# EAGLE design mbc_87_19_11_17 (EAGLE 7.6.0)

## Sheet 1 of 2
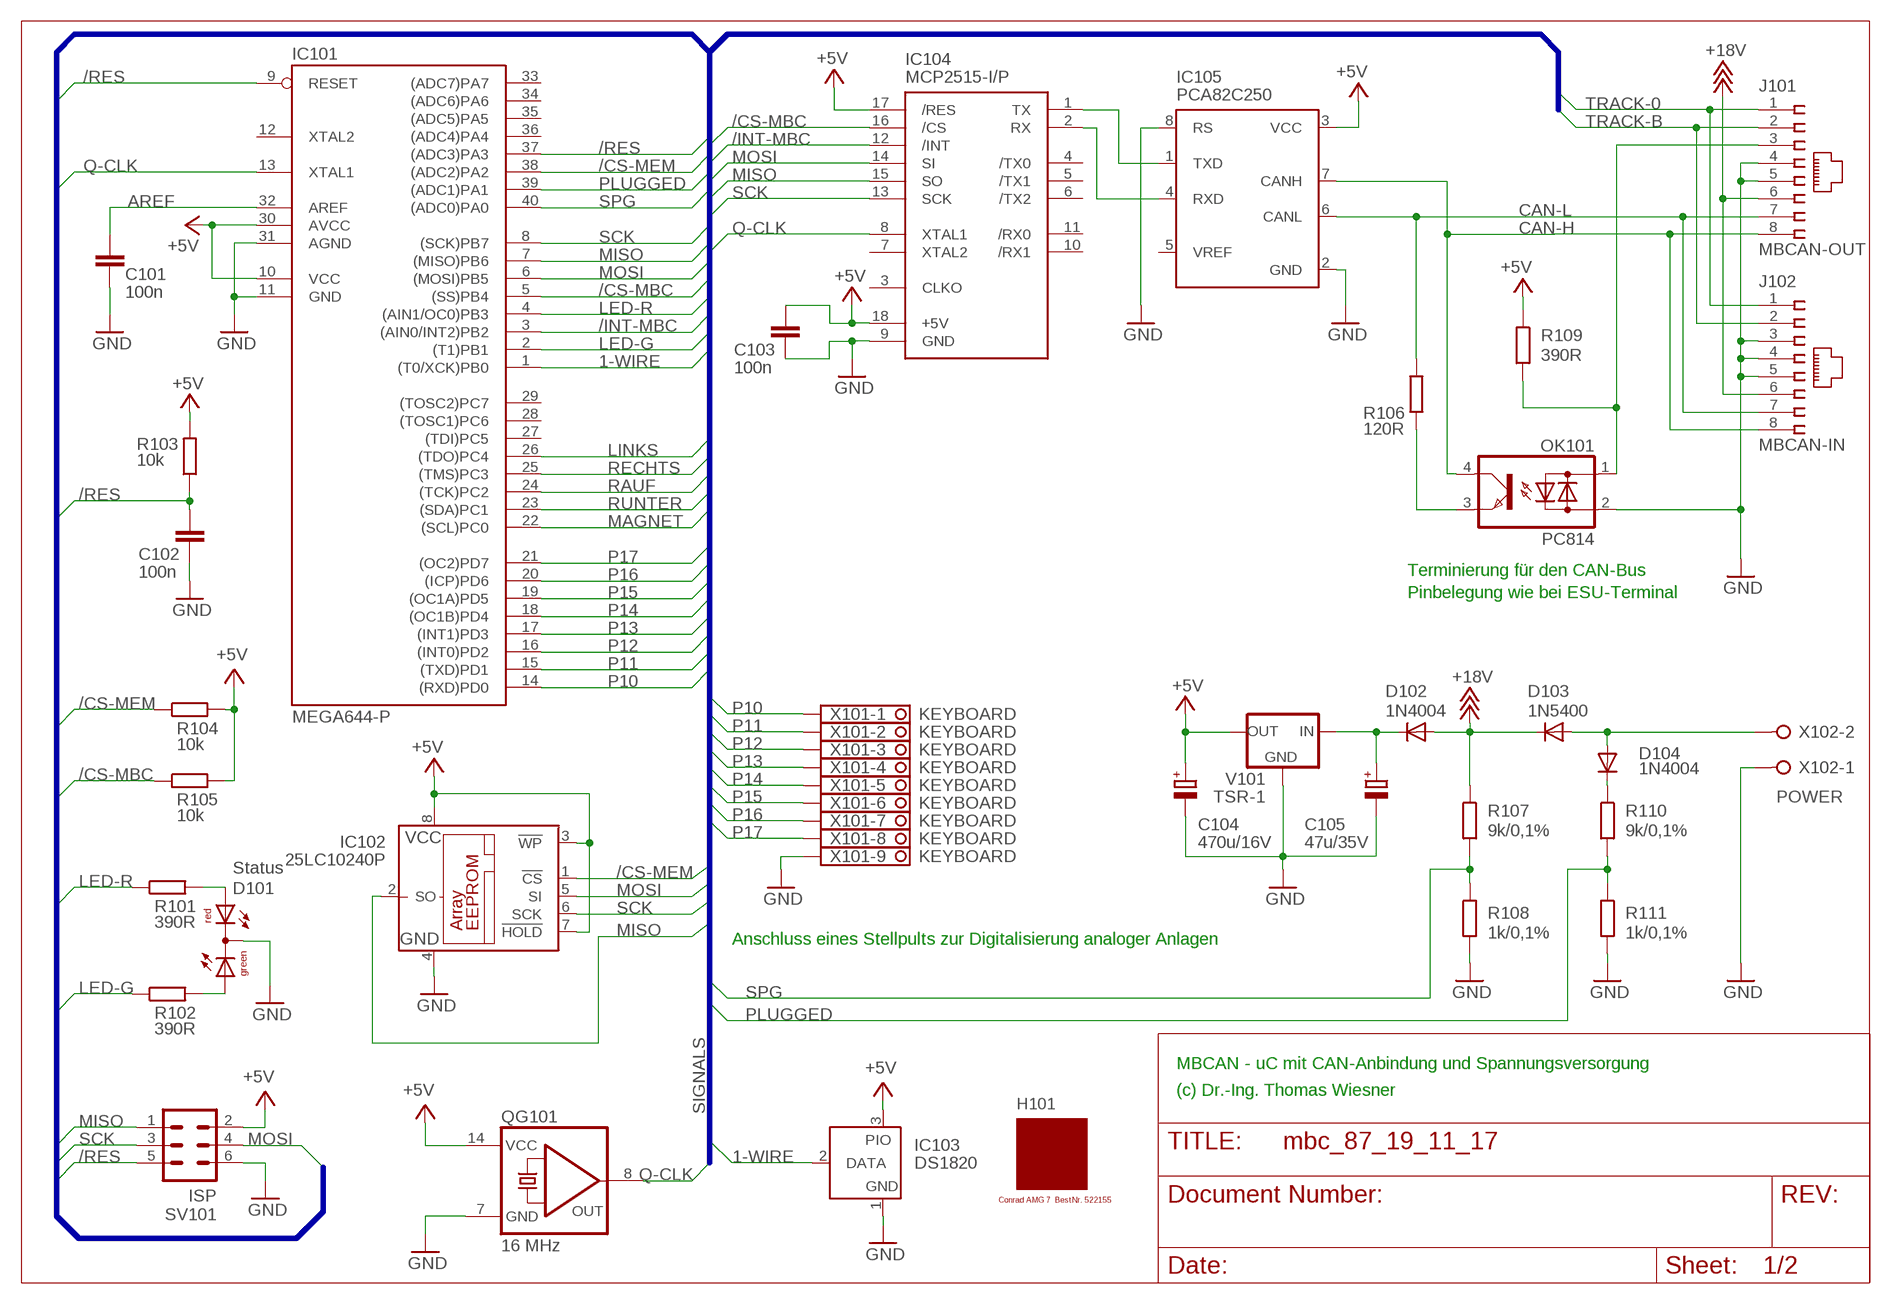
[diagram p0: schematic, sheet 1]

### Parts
C101  100n  C-EU025-025X050  [C025-025X050]
C102  100n  C-EU025-025X050  [C025-025X050]
C103  100n  C-EU025-025X050  [C025-025X050]
C104  470u/16V  CPOL-EUE3.5-8  [E3,5-8]
C105  47u/35V  CPOL-EUE2.5-7  [E2,5-7]
D101  Status  DUOLED5MM  [DUOLED5MM]
D102  1N4004  [DO41-10]
D103  1N5400  [DO201-15]
D104  1N4004  [DO41-10]
H101  MODULGEHÄUSE-AMG-7  [MODULGEHÄUSE-1]
IC101  MEGA644-P  MEGA323-P  [DIL40]
IC102  25LC10240P  25LC040P  [DIL8]
IC103  DS1820  DS2405  [TO92-]
IC104  MCP2515-I/P  MCP2510-I/P  [DIL18]
IC105  PCA82C250  [DIL08]
J101  MBCAN-OUT  215877-4  [215877-4]
J102  MBCAN-IN  215877-4  [215877-4]
OK101  PC814  [DIL04]
QG101  16 MHz  QG5860  [DIL14S]
R101  390R  R-EU_0207/10  [0207/10]
R102  390R  R-EU_0207/10  [0207/10]
R103  10k  R-EU_0207/10  [0207/10]
R104  10k  R-EU_0207/10  [0207/10]
R105  10k  R-EU_0207/10  [0207/10]
R106  120R  R-EU_0207/10  [0207/10]
R107  9k/0,1%  R-EU_0207/10  [0207/10]
R108  1k/0,1%  R-EU_0207/10  [0207/10]
R109  390R  R-EU_0207/10  [0207/10]
R110  9k/0,1%  R-EU_0207/10  [0207/10]
R111  1k/0,1%  R-EU_0207/10  [0207/10]
SV101  ISP  ML6  [ML6]
V101  TSR-1  [TRACO-TSR-1]
X101  KEYBOARD  1751316  [1751316]
X102  POWER  W237-02P  [W237-132]

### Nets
1-WIRE: IC101.1((T0/XCK)PB0) IC103.2(DATA)
+5V: C103.1 C104.+ IC101.10(VCC) IC101.30(AVCC) IC102.3(!WP) IC102.7(!HOLD) IC102.8(VCC) IC103.3(PIO) IC104.17(/RES) IC104.18(+5V) IC105.3(VCC) QG101.14(VCC) R103.2 R104.2 R105.2 R109.1 SV101.2 V101.OUT ; also sheet 2
+18V: D102.A D103.C J101.6 J102.6 R107.1
/CS-MBC: IC101.5((SS)PB4) IC104.16(/CS) R105.1
/CS-MEM: IC101.38((ADC2)PA2) IC102.1(!CS) R104.1
/INT-MBC: IC101.3((AIN0/INT2)PB2) IC104.12(/INT)
/RES: C102.1 IC101.9(RESET) IC101.37((ADC3)PA3) R103.1 SV101.5
AREF: C101.1 IC101.32(AREF)
CAN-H: IC105.7(CANH) J101.8 J102.8 OK101.4(C)
CAN-L: IC105.6(CANL) J101.7 J102.7 R106.2
GND: C101.2 C102.2 C103.2 C104.- C105.- D101.K(C) IC101.11(GND) IC101.31(AGND) IC102.4(GND) IC103.1(GND) IC104.9(GND) IC105.2(GND) IC105.8(RS) J101.4 J101.5 J102.3 J102.4 J102.5 OK101.2(AC2) QG101.7(GND) R108.2 R111.2 SV101.6 V101.GND X101.9 X102.1 ; also sheet 2
LED-G: IC101.2((T1)PB1) R102.1
LED-R: IC101.4((AIN1/OC0)PB3) R101.1
LINKS: IC101.26((TDO)PC4) ; also sheet 2
MAGNET: IC101.22((SCL)PC0) ; also sheet 2
MISO: IC101.7((MISO)PB6) IC102.2(SO) IC104.15(SO) SV101.1
MOSI: IC101.6((MOSI)PB5) IC102.5(SI) IC104.14(SI) SV101.4
N$1: IC104.1(TX) IC105.1(TXD)
N$2: IC104.2(RX) IC105.4(RXD)
N$3: OK101.3(E) R106.1
N$4: J101.3 OK101.1(AC1) R109.2
N$5: D104.C R110.1
N$6: C105.+ D102.C V101.IN
N$9: D101.AR R101.2
N$13: D101.AG R102.2
P10: IC101.14((RXD)PD0) X101.1
P11: IC101.15((TXD)PD1) X101.2
P12: IC101.16((INT0)PD2) X101.3
P13: IC101.17((INT1)PD3) X101.4
P14: IC101.18((OC1B)PD4) X101.5
P15: IC101.19((OC1A)PD5) X101.6
P16: IC101.20((ICP)PD6) X101.7
P17: IC101.21((OC2)PD7) X101.8
PLUGGED: IC101.39((ADC1)PA1) R110.2 R111.1
Q-CLK: IC101.13(XTAL1) IC104.8(XTAL1) QG101.8(OUT)
RAUF: IC101.24((TCK)PC2) ; also sheet 2
RECHTS: IC101.25((TMS)PC3) ; also sheet 2
RUNTER: IC101.23((SDA)PC1) ; also sheet 2
SCK: IC101.8((SCK)PB7) IC102.6(SCK) IC104.13(SCK) SV101.3
SPG: IC101.40((ADC0)PA0) R107.2 R108.1
TRACK-0: J101.1 J102.1
TRACK-B: J101.2 J102.2
V-NETZTEIL: D103.A D104.A X102.2
Unconnected: IC101.12(XTAL2) IC101.27((TDI)PC5) IC101.28((TOSC1)PC6) IC101.29((TOSC2)PC7) IC101.33((ADC7)PA7) IC101.34((ADC6)PA6) IC101.35((ADC5)PA5) IC101.36((ADC4)PA4) IC104.3(CLKO) IC104.4(/TX0) IC104.5(/TX1) IC104.6(/TX2) IC104.7(XTAL2) IC104.10(/RX1) IC104.11(/RX0) IC105.5(VREF)

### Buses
SIGNALS

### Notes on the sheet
- Terminierung für den CAN-Bus
- Pinbelegung wie bei ESU-Terminal
- Anschluss eines Stellpults zur Digitalisierung analoger Anlagen
- MBCAN - uC mit CAN-Anbindung und Spannungsversorgung
- (c) Dr.-Ing. Thomas Wiesner

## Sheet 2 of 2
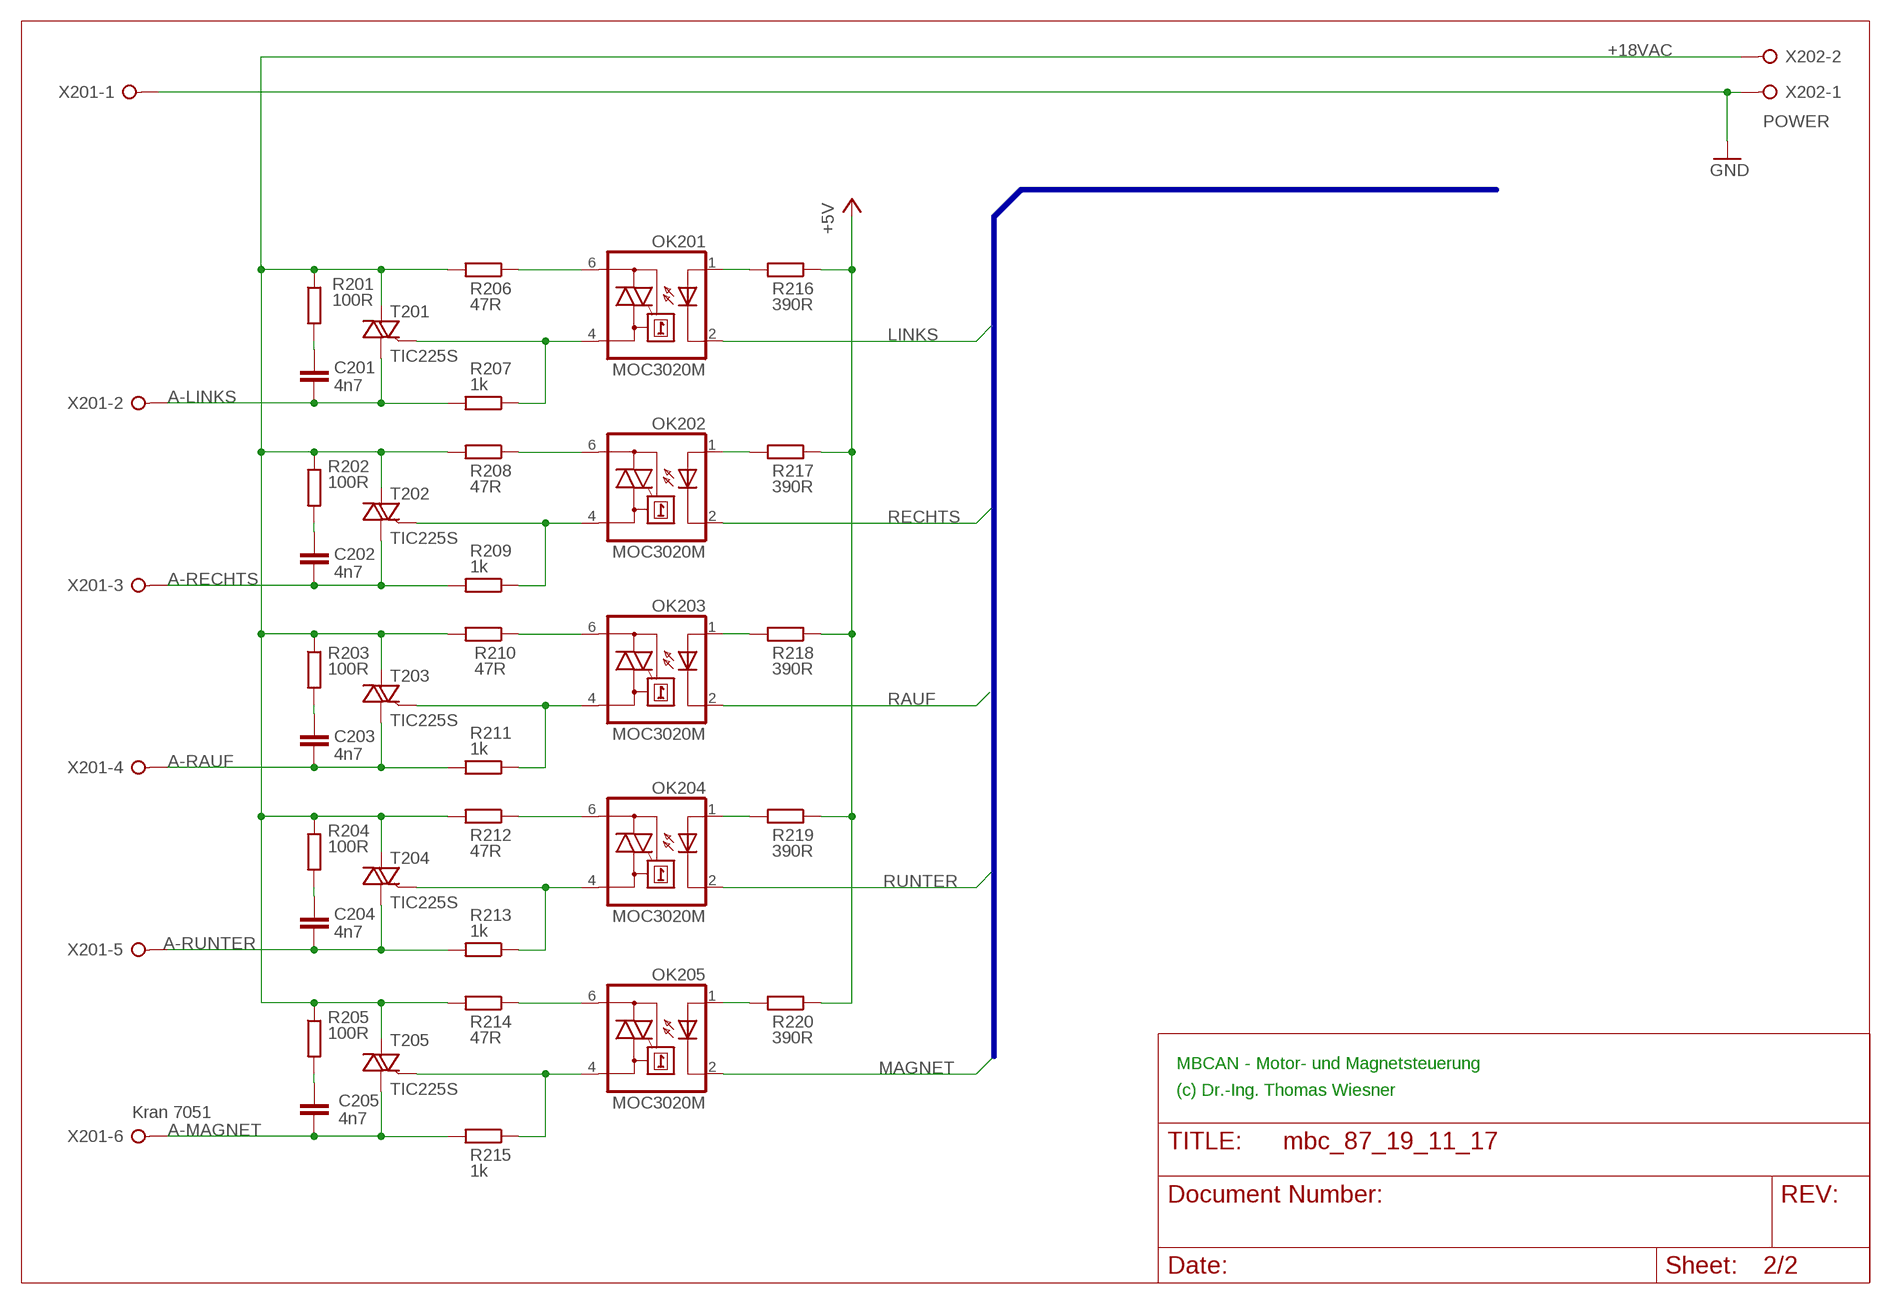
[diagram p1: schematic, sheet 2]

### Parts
C201  4n7  C-EU025-025X050  [C025-025X050]
C202  4n7  C-EU025-025X050  [C025-025X050]
C203  4n7  C-EU025-025X050  [C025-025X050]
C204  4n7  C-EU025-025X050  [C025-025X050]
C205  4n7  C-EU025-025X050  [C025-025X050]
OK201  MOC3020M  [DIL06]
OK202  MOC3020M  [DIL06]
OK203  MOC3020M  [DIL06]
OK204  MOC3020M  [DIL06]
OK205  MOC3020M  [DIL06]
R201  100R  R-EU_0207/10  [0207/10]
R202  100R  R-EU_0207/10  [0207/10]
R203  100R  R-EU_0207/10  [0207/10]
R204  100R  R-EU_0207/10  [0207/10]
R205  100R  R-EU_0207/10  [0207/10]
R206  47R  R-EU_0207/10  [0207/10]
R207  1k  R-EU_0207/10  [0207/10]
R208  47R  R-EU_0207/10  [0207/10]
R209  1k  R-EU_0207/10  [0207/10]
R210  47R  R-EU_0207/10  [0207/10]
R211  1k  R-EU_0207/10  [0207/10]
R212  47R  R-EU_0207/10  [0207/10]
R213  1k  R-EU_0207/10  [0207/10]
R214  47R  R-EU_0207/10  [0207/10]
R215  1k  R-EU_0207/10  [0207/10]
R216  390R  R-EU_0207/10  [0207/10]
R217  390R  R-EU_0207/10  [0207/10]
R218  390R  R-EU_0207/10  [0207/10]
R219  390R  R-EU_0207/10  [0207/10]
R220  390R  R-EU_0207/10  [0207/10]
T201  TIC225S  [TO220DS]
T202  TIC225S  [TO220DS]
T203  TIC225S  [TO220DS]
T204  TIC225S  [TO220DS]
T205  TIC225S  [TO220DS]
X201  Kran 7051  W237-06P  [W237-6P]
X202  POWER  W237-02P  [W237-132]

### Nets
+5V: R216.1 R217.1 R218.1 R219.1 R220.1 ; also sheet 1
+18VAC: R201.1 R202.1 R203.1 R204.1 R205.1 R206.2 R208.2 R210.2 R212.2 R214.2 T201.A2 T202.A2 T203.A2 T204.A2 T205.A2 X202.2
A-LINKS: C201.2 R207.2 T201.A1 X201.2
A-MAGNET: C205.2 R215.2 T205.A1 X201.6
A-RAUF: C203.2 R211.2 T203.A1 X201.4
A-RECHTS: C202.2 R209.2 T202.A1 X201.3
A-RUNTER: C204.2 R213.2 T204.A1 X201.5
GND: X201.1 X202.1 ; also sheet 1
LINKS: OK201.2(C) ; also sheet 1
MAGNET: OK205.2(C) ; also sheet 1
N$7: OK201.1(A) R216.2
N$10: OK201.4(A1) R207.1 T201.G
N$11: OK201.6(A2) R206.1
N$12: OK202.1(A) R217.2
N$15: C201.1 R201.2
N$17: OK202.4(A1) R209.1 T202.G
N$18: OK202.6(A2) R208.1
N$20: C202.1 R202.2
N$21: OK203.1(A) R218.2
N$23: OK203.4(A1) R211.1 T203.G
N$24: OK203.6(A2) R210.1
N$26: C203.1 R203.2
N$27: OK204.1(A) R219.2
N$29: OK204.4(A1) R213.1 T204.G
N$30: OK204.6(A2) R212.1
N$32: C204.1 R204.2
N$33: OK205.1(A) R220.2
N$35: OK205.4(A1) R215.1 T205.G
N$36: OK205.6(A2) R214.1
N$38: C205.1 R205.2
RAUF: OK203.2(C) ; also sheet 1
RECHTS: OK202.2(C) ; also sheet 1
RUNTER: OK204.2(C) ; also sheet 1

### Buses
B$1

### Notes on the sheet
- MBCAN - Motor- und Magnetsteuerung
- (c) Dr.-Ing. Thomas Wiesner

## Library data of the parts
C101-C103 = rcl:C-EU: CAPACITOR, European symbol
C104 C105 = rcl:CPOL-EU: POLARIZED CAPACITOR, European symbol
C201-C205 = resistor:C-EU: CAPACITOR, European symbol
D101 = led:DUOLED5MM: DUO LED 2 colors, 5 mm, round
D102 D104 = diode:1N4004: DIODE
D103 = diode:1N5400: DIODE
H101 = mbc:MODULGEHÄUSE-AMG-7: Gehäuse
IC101 = atmel:MEGA323-P: MICROCONTROLLER 32 Kbytes FLASH 2 Kbytes SRAM 1 Kbytes EEPROM USART 8-channel 10 bit ADC Source: avr.lbr; OC_FARNELL: unknown; OC_NEWARK: unknown
IC102 = microchip:25*: Serial EEPROM 4K/ 8K , SPI bus; MF: MICROCHIP; MPN: 25LC040/P; OC_FARNELL: 9758100; OC_NEWARK: 96K4091
IC103 = maxim:DS2405: Addressable Switch DALLAS Semiconductor; MF: DALLAS SEMICONDUCTOR; MPN: DS2405; OC_FARNELL: 1188025; OC_NEWARK: 06F4645
IC104 = mbc:MCP2510: BASIC-CAN 2.0a Controller Stand-alone CAN controller von Microchip
IC105 = micro-philips:PCA82C250: CAN CONTROLLER INTERFACE; OC_FARNELL: 3692358; OC_NEWARK: unknown
J101 J102 = con-amp:215877-4: AMP connector
OK101 = optocoupler:PC814: SHARP OPTO COUPLER; OC_FARNELL: 9707662; OC_NEWARK: unknown
OK201-OK205 = optocoupler:MOC30*M: RANDOM-PHASE OPTOISOLATORS TRIAC DRIVER OUTPUT Source: http://www.fairchildsemi.com MOC3020-M.pdf; MF: FAIRCHILD SEMICONDUCTOR; MPN: MOC3020-M; OC_FARNELL: 1505425; OC_NEWARK: 72K8895
QG101 = crystal:QG5860: CRYSTAL RESONATOR; OC_FARNELL: unknown; OC_NEWARK: unknown
R101-R111 R201-R220 = resistor:R-EU_: RESISTOR, European symbol
SV101 = con-ml:ML6: HARTING; OC_FARNELL: unknown; OC_NEWARK: unknown
T201-T205 = triac:TIC225S: TRIAC
V101 = mbc:TSR-1: Spannungsregler Hersteller: TRACO Typ: TSR-1 5V: TSR 1-2450 Spg: 5V Strom: 1A Reichelt TSR 1-2450
X101 = con-phoenix-350:1751316: MKDS 1/ 9-3,5 Printklemme Nennstrom: 10 A Bemessungsspannung: 160 V Raster: 3,5 mm Polzahl: 9 Montageart: Löten Anschlussart: Schraubanschluss Anschlussrichtung vom Leiter zur Platine: 0° Source: http://eshop.phoenixcontact.com .. 1751316.pdf; OC_FARNELL: unknown; OC_NEWARK: unknown
X102 X202 = con-wago-508:W237-02P: WAGO SREW CLAMP; OC_FARNELL: unknown; OC_NEWARK: unknown
X201 = con-wago-508:W237-06P: WAGO SREW CLAMP; OC_FARNELL: unknown; OC_NEWARK: unknown

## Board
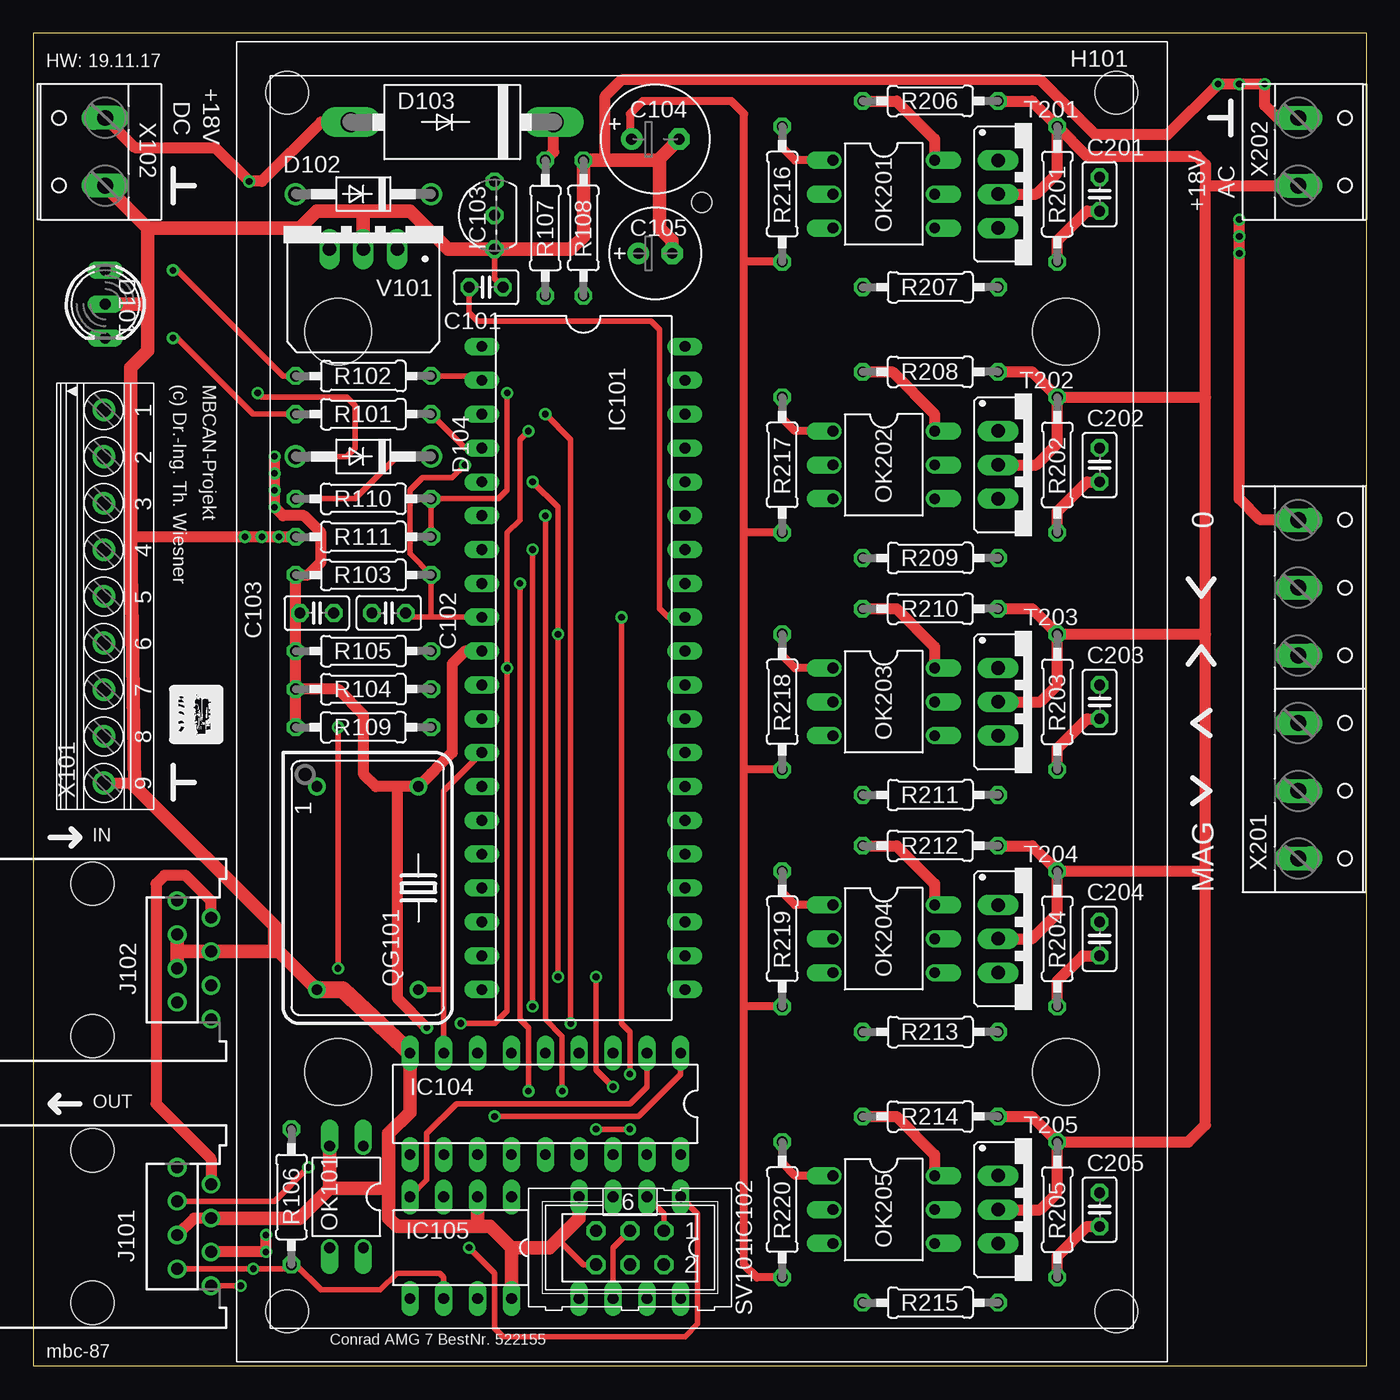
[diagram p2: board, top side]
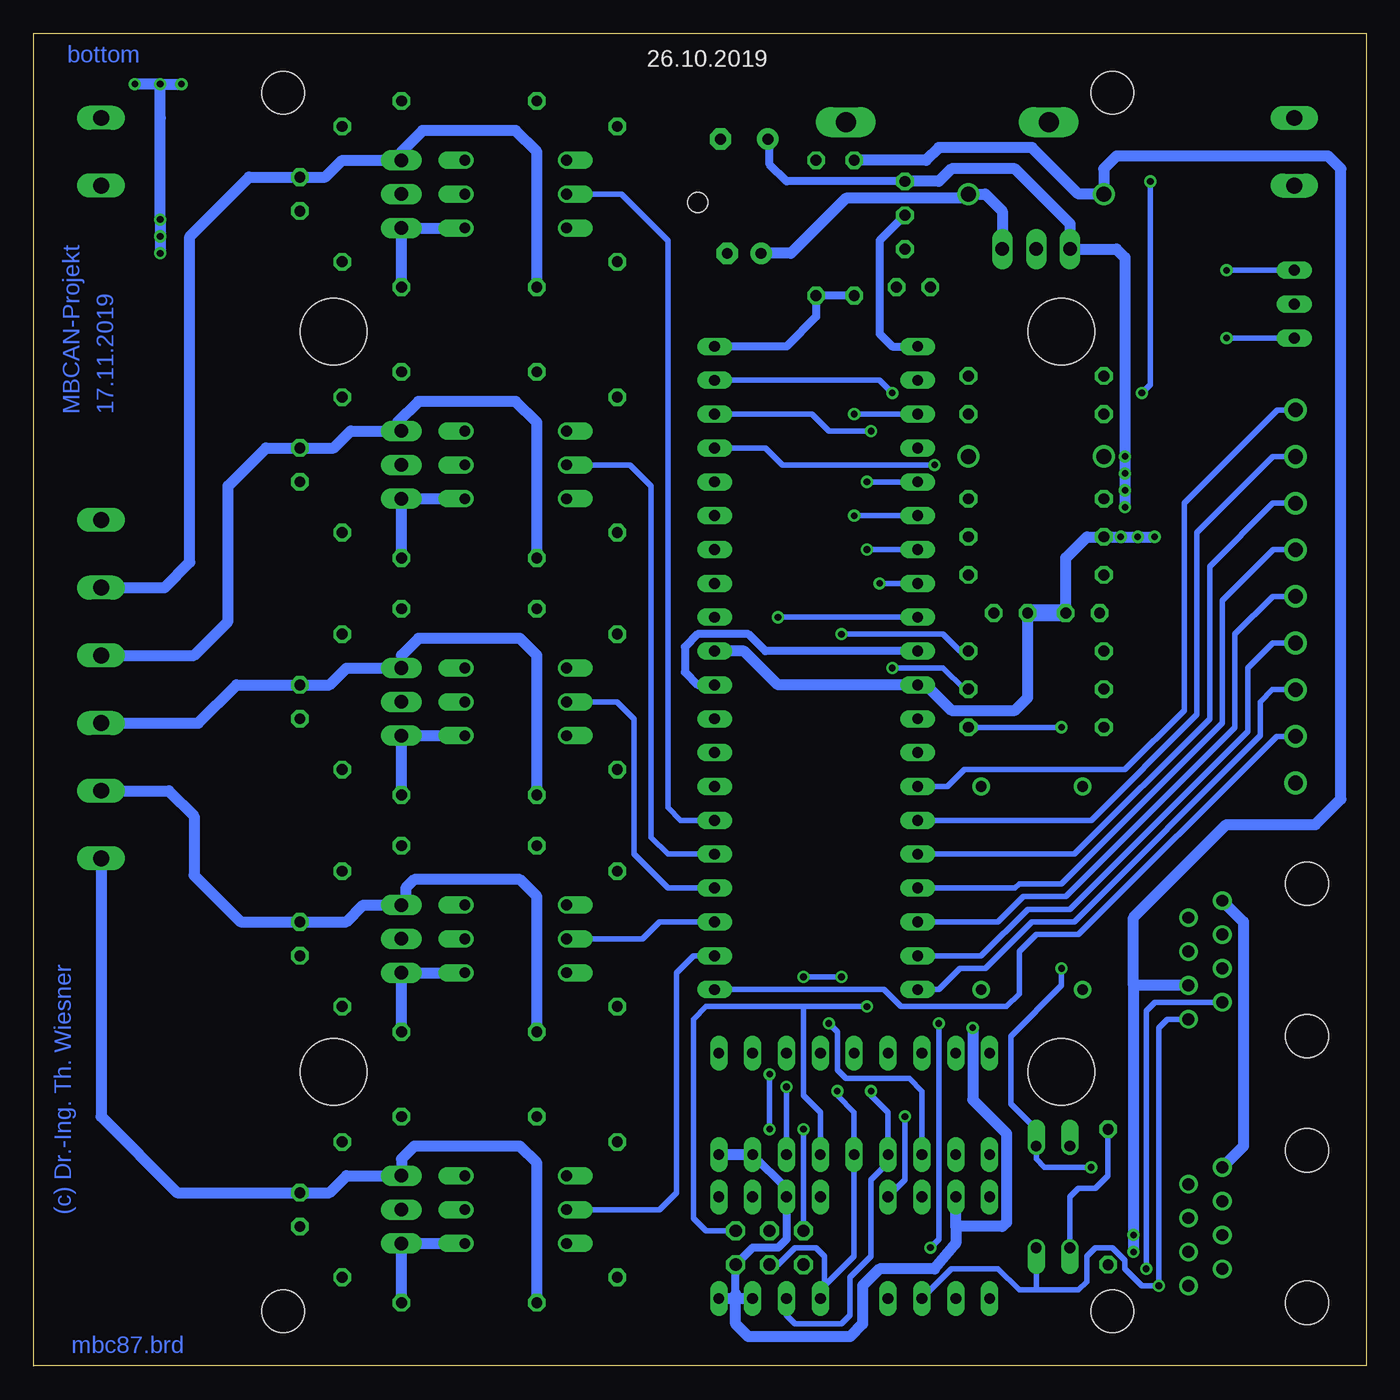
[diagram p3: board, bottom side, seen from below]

Size 100.01 x 100.01 mm. Coordinates in mm from the lower left corner, seen from the top.
Outline: 100,0.02 0,0.02 0,100.01 100,100.01
Outline: 100.01,100.01 100.01,0
Copper layers (1*16): Top 0.035mm / dielectric 1.5mm / Bottom 0.035mm
Design rules "default *": minimum track width 10mil, minimum drill 0.5mm, track to track 8mil, track to pad 8mil, pad to pad 8mil, via to via 8mil, smd to smd 8mil, copper to edge 40mil, drill to drill 8mil, minimum pad ring 10mil, minimum via ring 8mil, stop-mask expansion 4mil, vias tented up to drill 0mil, thermal gap 10mil

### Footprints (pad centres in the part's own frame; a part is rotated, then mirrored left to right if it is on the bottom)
C025-025X050 = drill 0.813 octagon: 1 -1.27,0; 2 1.27,0
E3,5-8 = drill 0.813 pad 1.6: + -1.778,0 | drill 0.813 pad 1.6 octagon: - 1.778,0
E2,5-7 = drill 0.813 pad 1.6: + -1.27,0 | drill 0.813 pad 1.6 octagon: - 1.27,0
DUOLED5MM = drill 0.813 long: AG -2.54,0; AR 2.54,0; K 0,0
DO41-10 = drill 1.118: A 5.08,0; C -5.08,0
DO201-15 = drill 1.499 long: A 7.62,0; C -7.62,0
MODULGEHÄUSE-1 = hole 3.2: -45.72,-31.115; -45.72,31.115; 45.72,31.115; 45.72,-31.115 | hole 5: -27.781,-27.305; 27.781,-27.305; -27.781,27.305; 27.781,27.305 | hole 1.5: -37.465,0
DIL40 = drill 0.813 long: 1 -24.13,-7.62; 2 -21.59,-7.62; 3 -19.05,-7.62; 4 -16.51,-7.62; 5 -13.97,-7.62; 6 -11.43,-7.62; 7 -8.89,-7.62; 8 -6.35,-7.62; 9 -3.81,-7.62; 10 -1.27,-7.62; 11 1.27,-7.62; 12 3.81,-7.62; 13 6.35,-7.62; 14 8.89,-7.62; 15 11.43,-7.62; 16 13.97,-7.62; 17 16.51,-7.62; 18 19.05,-7.62; 19 21.59,-7.62; 20 24.13,-7.62; 21 24.13,7.62; 22 21.59,7.62; 23 19.05,7.62; 24 16.51,7.62; 25 13.97,7.62; 26 11.43,7.62; 27 8.89,7.62; 28 6.35,7.62; 29 3.81,7.62; 30 1.27,7.62; 31 -1.27,7.62; 32 -3.81,7.62; 33 -6.35,7.62; 34 -8.89,7.62; 35 -11.43,7.62; 36 -13.97,7.62; 37 -16.51,7.62; 38 -19.05,7.62; 39 -21.59,7.62; 40 -24.13,7.62
DIL8 = drill 0.813 long: 1 -3.81,-3.81; 2 -1.27,-3.81; 3 1.27,-3.81; 4 3.81,-3.81; 5 3.81,3.81; 6 1.27,3.81; 7 -1.27,3.81; 8 -3.81,3.81
TO92- = drill 0.813 octagon: 1 -2.54,0; 2 0,0; 3 2.54,0
DIL18 = drill 0.813 long: 1 -10.16,-3.81; 2 -7.62,-3.81; 3 -5.08,-3.81; 4 -2.54,-3.81 | drill 0.8 long: 5 0,-3.81; 6 2.54,-3.81; 7 5.08,-3.81; 8 7.62,-3.81; 9 10.16,-3.81; 10 10.16,3.81; 11 7.62,3.81; 12 5.08,3.81; 13 2.54,3.81; 14 0,3.81; 15 -2.54,3.81; 16 -5.08,3.81; 17 -7.62,3.81; 18 -10.16,3.81
DIL08 = drill 0.813 long: 1 -3.81,-3.81; 2 -1.27,-3.81; 3 1.27,-3.81; 4 3.81,-3.81; 5 3.81,3.81; 6 1.27,3.81; 7 -1.27,3.81; 8 -3.81,3.81
215877-4 = drill 0.889: 1 -4.445,6.35; 2 -3.175,8.89; 3 -1.905,6.35; 4 -0.635,8.89; 5 0.635,6.35; 6 1.905,8.89; 7 3.175,6.35; 8 4.445,8.89 | hole 3.251: -5.715,0; 5.715,0
DIL04 = drill 0.813 offset: 1 -1.27,-3.81; 2 1.27,-3.81; 3 1.27,3.81; 4 -1.27,3.81
DIL06 = drill 0.813 offset: 1 -2.54,-3.81; 2 0,-3.81; 3 2.54,-3.81; 4 2.54,3.81; 5 0,3.81; 6 -2.54,3.81
DIL14S = drill 0.813: 1 -7.62,-3.81; 7 7.62,-3.81; 8 7.62,3.81; 14 -7.62,3.81
0207/10 = drill 0.813 octagon: 1 -5.08,0; 2 5.08,0
ML6 = drill 0.914 octagon: 1 -2.54,-1.27; 2 -2.54,1.27; 3 0,-1.27; 4 0,1.27; 5 2.54,-1.27; 6 2.54,1.27
TO220DS = drill 1.016 long: A1 -2.54,-2.54; A2 0,-2.54; G 2.54,-2.54
TRACO-TSR-1 = drill 1.016 long: GND 0,2.54; IN -2.54,2.54; OUT 2.54,2.54
1751316 = drill 1.1 pad 1.7: 1 -13.973,-0.1; 2 -10.473,-0.1; 3 -6.973,-0.1; 4 -3.473,-0.1; 5 0.028,-0.1; 6 3.527,-0.1; 7 7.027,-0.1; 8 10.527,-0.1; 9 14.027,-0.1
W237-132 = drill 1.194 long: 1 -2.54,-0.635; 2 2.54,-0.635
W237-6P = drill 1.194 long: 1 -12.7,-0.635; 2 -7.62,-0.635; 3 -2.54,-0.635; 4 2.54,-0.635; 5 7.62,-0.635; 6 12.7,-0.635

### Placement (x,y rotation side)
C101  33.97,80.96 0 top
C102  26.67,56.52 180 top
C103  21.27,56.52 0 top
C104  46.67,92.08 0 top
C105  46.67,83.5 0 top
C201  80.01,87.95 90 top
C202  80.01,67.63 90 top
C203  80.01,49.85 90 top
C204  80.01,32.07 90 top
C205  80.01,11.75 90 top
D101  5.4,79.69 270 top
D102  24.77,87.95 180 top
D103  31.43,93.34 180 top
D104  24.77,68.26 180 top
H101  50.16,49.85 270 top
IC101  41.27,52.39 270 top
IC102  44.77,8.89 180 top
IC103  34.61,86.36 90 top
IC104  38.42,19.68 180 top
IC105  32.07,8.89 180 top
J101  4.45,10.48 270 top
J102  4.45,30.48 270 top
OK101  23.5,12.7 180 top
OK201  63.82,87.95 270 top
OK202  63.82,67.63 270 top
OK203  63.82,49.85 270 top
OK204  63.82,32.07 270 top
OK205  63.82,11.75 270 top
QG101  25.08,35.88 270 top
R101  24.77,71.44 180 top
R102  24.77,74.3 180 top
R103  24.77,59.37 180 top
R104  24.77,50.8 180 top
R105  24.77,53.66 180 top
R106  19.37,12.7 270 top
R107  38.42,85.41 270 top
R108  41.27,85.41 90 top
R109  24.77,47.94 0 top
R110  24.77,65.09 0 top
R111  24.77,62.23 180 top
R201  76.83,87.95 270 top
R202  76.83,67.63 270 top
R203  76.83,49.85 270 top
R204  76.83,32.07 270 top
R205  76.83,11.75 270 top
R206  67.31,94.93 0 top
R207  67.31,80.96 180 top
R208  67.31,74.61 0 top
R209  67.31,60.64 180 top
R210  67.31,56.83 0 top
R211  67.31,42.86 180 top
R212  67.31,39.05 0 top
R213  67.31,25.08 180 top
R214  67.31,18.73 0 top
R215  67.31,4.76 180 top
R216  56.2,87.95 90 top
R217  56.2,67.63 90 top
R218  56.2,49.85 90 top
R219  56.2,32.07 90 top
R220  56.2,11.75 90 top
SV101  44.77,8.89 180 top
T201  74.93,87.95 270 top
T202  74.93,67.63 270 top
T203  74.93,49.85 270 top
T204  74.93,32.07 270 top
T205  74.93,11.75 270 top
V101  24.77,86.36 180 top
X101  5.4,57.78 270 top
X102  4.76,91.12 90 top
X201  95.57,50.8 270 top
X202  95.57,91.12 270 top

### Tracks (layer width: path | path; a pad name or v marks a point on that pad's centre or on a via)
1-WIRE
  Bottom 0.61: IC103.2 36.51,84.45 36.51,77.47 35.56,76.52 IC101.1
+5V  (via drill 0.5)
  Top 0.61: R220.1 54.29,6.67 53.34,7.62 53.34,26.99 | 53.34,26.99 53.34,44.77 | 53.34,44.77 53.34,62.55 | 53.34,62.55 53.34,82.87 | 53.34,82.87 53.34,93.98 52.39,94.93 45.72,94.93 44.77,93.98 44.77,92.2 C104.+ | R216.1 53.34,82.87 | R217.1 53.34,62.55 | R218.1 53.34,44.77 | R219.1 53.34,26.99
  Top 0.813: IC101.10 32.38,53.66 31.43,52.7 31.43,46.04 QG101.14 | v29.53,25.4 27.3,27.62 27.3,43.5 | v18.1,68.26 v18.1,66.99 v18.1,65.72 v18.1,64.45 18.73,63.82 20.32,63.82 21.59,62.55 21.59,60.33 20.64,59.37 R103.2 19.68,56.52 | QG101.14 29.84,44.45 | QG101.14 27.3,43.5 | 27.3,43.5 25.72,43.5 24.77,44.45 24.77,48.9 22.86,50.8 R104.2 | R109.1 R104.2 | R104.2 R105.2 19.68,56.52 | C103.1 19.68,56.52
  Bottom 0.406: IC102.3 43.5,13.34
  Bottom 0.61: IC101.10 45.09,53.66 46.35,54.93 50.16,54.93 51.12,53.98 51.12,52.07 50.16,51.12 IC101.30 | IC102.3 43.5,9.53 44.13,8.89 46.04,8.89 SV101.2 47.31,5.4 | 43.5,13.34 IC104.17 | IC103.3 43.5,88.9 44.77,90.17 44.77,91.95 C104.+
  Bottom 0.813: v18.1,64.45 v18.1,65.72 v18.1,66.99 v18.1,68.26 18.1,83.19 18.73,83.82 V101.OUT 22.23,85.72 26.35,89.85 31.11,89.85 32.07,88.9 IC103.3 | 30.8,10.48 30.8,9.21 32.38,7.3 36.51,7.3 37.78,6.03 37.78,3.17 38.73,2.22 46.35,2.22 47.31,3.17 47.31,5.08 | 30.8,10.48 27.3,10.48 26.99,10.79 26.99,17.46 29.53,20 v29.53,25.4 | 30.8,10.48 IC105.3 | 47.31,5.08 46.99,5.08 | 46.99,5.08 IC102.7 | IC102.8 47.31,5.08 | IC104.17 IC104.18 | 47.31,5.4 46.99,5.08
+18V  (via drill 0.5)
  Top 0.813: D103.C 39.05,91.12 R107.1 | J101.6 v17.46,8.57 v17.46,9.84
  Bottom 0.406: 19.68,88.27 D102.A
  Bottom 0.813: R107.1 33.02,90.49 32.07,91.44 25.08,91.44 21.59,87.95 D102.A | J102.6 17.46,28.57 | 17.46,28.57 v17.46,9.84 v17.46,8.57 | 17.46,28.57 17.46,33.66 10.48,40.64 3.81,40.64 1.91,42.55 1.91,89.85 2.86,90.81 18.73,90.81 19.68,89.85 19.68,88.27
+18VAC
  Top 0.813: T205.A2 75.56,11.75 76.83,13.02 R205.1 | R205.1 86.68,16.83 87.95,18.1 87.95,37.15 | 87.95,37.15 87.95,54.93 | 87.95,54.93 87.95,72.71 | 87.95,72.71 87.95,88.58 | 87.95,88.58 X202.2 | R201.1 79.06,90.81 87.31,90.81 87.95,90.17 87.95,88.58 | R206.2 74.93,94.93 R201.1 | R202.1 87.95,72.71 | R203.1 87.95,54.93 | R204.1 87.95,37.15 | R212.2 74.93,39.05 R204.1 | R214.2 74.93,18.73 R205.1 | R210.2 74.93,56.83 R203.1 | R208.2 74.93,74.61 R202.1 | T201.A2 75.25,87.95 76.83,89.53 R201.1 | T202.A2 75.25,67.63 76.83,69.22 R202.1 | T203.A2 75.56,49.85 76.83,51.12 R203.1 | T204.A2 74.93,32.07 76.83,33.97 R204.1
/CS-MBC  (via drill 0.5)
  Top 0.406: v37.47,66.36 39.37,64.45 v39.37,54.93 v39.37,29.21 | v43.5,20.95 42.23,22.23 v42.23,29.21
  Bottom 0.406: IC101.5 v37.47,66.36 | v39.37,29.21 v42.23,29.21 | v43.5,20.95 IC104.16 | R105.1 30.48,53.66 31.75,54.93 v39.37,54.93
/CS-MEM  (via drill 0.5)
  Top 0.406: v32.7,8.89 34.61,6.99 34.61,2.86 35.24,2.22 48.9,2.22 49.85,3.17 49.85,11.43 IC102.1 | v37.15,70.17 36.51,69.53 36.51,63.5 35.56,62.55 v35.56,52.39 35.56,26.67 34.61,25.72 v32.07,25.72
  Bottom 0.406: IC101.38 41.59,71.44 40.32,70.17 v37.15,70.17 | v32.7,8.89 32.07,9.53 v32.07,25.72 | R104.1 30.16,50.8 31.75,52.39 v35.56,52.39
/INT-MBC  (via drill 0.5)
  Top 0.406: v40.32,25.72 40.32,69.53 v38.42,71.44
  Bottom 0.406: IC104.12 33.34,20.64 34.29,21.59 39.05,21.59 39.69,22.23 39.69,25.08 v40.32,25.72 | v38.42,71.44 IC101.3
/RES  (via drill 0.5)
  Top 0.406: 29.84,56.2 28.26,56.2 C102.1 | 29.84,56.2 IC101.9 | v32.38,67.63 31.43,66.67 29.21,66.67 28.26,65.72 28.26,60.96 R103.1 29.84,56.2 | v44.13,56.2 44.13,25.72 44.77,25.08 v44.77,21.91 | v44.77,17.78 v42.23,17.78
  Bottom 0.406: IC101.37 45.09,68.9 43.81,67.63 v32.38,67.63 | IC101.9 v44.13,56.2 | v44.77,21.91 v44.77,17.78 | v42.23,17.78 SV101.5
A-LINKS
  Bottom 0.813: X201.2 90.17,58.42 88.27,60.33 88.27,84.77 83.82,89.22 C201.2 78.11,89.22 76.83,90.49 T201.A1 72.39,91.12 70.8,92.71 63.82,92.71 62.23,91.12 R207.2
A-MAGNET
  Bottom 0.813: X201.6 94.93,18.73 89.22,13.02 C205.2 77.79,13.02 76.52,14.29 T205.A1 72.39,15.56 71.44,16.51 63.5,16.51 62.23,15.24 R215.2
A-RAUF
  Bottom 0.813: X201.4 87.63,48.26 84.77,51.12 C203.2 77.79,51.12 76.52,52.39 T203.A1 72.39,53.34 71.12,54.61 63.5,54.61 62.23,53.34 R211.2
A-RECHTS
  Bottom 0.813: X201.3 87.95,53.34 85.41,55.88 85.41,66.04 82.55,68.9 C202.2 77.47,68.9 76.2,70.17 T202.A1 72.71,70.48 72.71,70.8 71.12,72.39 63.82,72.39 62.23,70.8 R209.2
A-RUNTER
  Bottom 0.813: X201.5 89.85,43.18 87.95,41.27 87.95,36.83 84.45,33.34 C204.2 76.52,33.34 75.25,34.61 T204.A1 72.07,34.92 72.07,35.88 71.44,36.51 63.5,36.51 62.23,35.24 R213.2
AREF
  Top 0.406: IC101.32 47.62,56.2 46.99,56.83 46.99,77.79 46.35,78.42 33.34,78.42 32.7,79.06 C101.1
CAN-H  (via drill 0.5)
  Top 0.406: v15.56,6.03 J101.8
  Bottom 0.406: J102.8 14.92,26.04 15.56,25.4 v15.56,6.03 16.83,6.03 18.1,7.3 18.1,7.94 19.05,8.89 20.32,8.89 20.95,8.26 20.95,6.35 21.59,5.71 24.77,5.71 | 24.77,5.71 OK101.4 | IC105.7 31.11,7.3 27.62,7.3 26.04,5.71 24.77,5.71
CAN-L  (via drill 0.5)
  Top 0.406: IC105.6 30.8,6.67 30.48,6.99 27.3,6.99 26.04,5.71 21.59,5.71 19.68,7.62 R106.2 19.05,7.3 v16.51,7.3 J101.7
  Bottom 0.406: J102.7 15.88,27.3 16.51,26.67 v16.51,7.3
GND  (via drill 0.5)
  Top 0.406: C104.- 48.45,91.95 46.99,90.49 | IC103.1 34.61,81.6 C101.2 | SV101.6 41.27,7.62 39.37,9.53
  Top 0.813: R111.2 v18.41,62.23 v17.14,62.23 v15.88,62.23 7.3,62.23 | J101.4 12.06,11.11 J101.5 | 18.1,31.11 18.41,31.11 | X101.9 7.88,43.76 arc90 7.62,43.5 | X202.1 93.34,93.66 92.39,94.61 v92.39,96.2 v90.49,96.2 v88.9,96.2 85.09,92.39 79.69,92.39 75.56,96.52 44.13,96.52 42.86,95.25 42.86,90.49 | X201.1 92.08,63.5 90.49,65.09 v90.49,83.5 v90.49,84.77 v90.49,86.04
  Top 1.016: C104.- 46.86,90.49 42.86,90.49 R108.2 41.27,84.77 40.32,83.82 IC103.1 31.11,83.82 28.26,86.68 24.77,86.68 | 24.77,86.68 V101.GND | 24.77,86.68 21.27,86.68 20,85.41 8.57,85.41 | 46.99,90.49 46.99,85.41 47.94,84.45 C105.- | X102.1 8.57,85.41 | 8.57,85.41 8.57,79.69 | D101.K 8.57,79.69 | 8.57,79.69 8.57,76.2 7.3,74.93 7.3,62.23 7.62,43.5 18.1,33.02 18.1,31.11 J102.4 10.79,31.11 | 10.79,31.11 J102.3 | 10.79,31.11 J102.5 | 18.41,31.11 QG101.7 | J101.4 20,11.11 22.23,13.34 | IC104.9 28.26,19.05 26.67,17.46 26.67,13.34 | 26.67,13.34 26.67,11.11 27.3,10.48 33.34,10.48 | 33.34,10.48 IC105.2 | IC105.8 35.88,8.89 | 35.88,8.89 34.29,10.48 33.34,10.48 | OK101.2 22.23,13.34 | 22.23,13.34 26.67,13.34 | 35.88,8.89 38.73,8.89 39.37,9.53 40.96,11.11 IC102.4
  Top 1.27: IC104.9 23.18,28.26 QG101.7
  Bottom 0.813: IC101.31 46.67,53.66 44.13,51.12 IC101.11 33.02,51.12 31.11,49.21 26.35,49.21 25.4,50.16 C102.2 | C103.2 22.54,60.64 20.95,62.23 R111.2 v18.41,62.23 v17.14,62.23 v15.88,62.23 | v90.49,83.5 v90.49,84.77 v90.49,86.04 90.49,93.66 | 90.49,93.66 v90.49,96.2 | v90.49,96.2 v92.39,96.2 | 90.49,93.66 v90.49,96.2 | v90.49,96.2 v88.9,96.2
  Bottom 1.27: C103.2 C102.2
LED-G
  Top 0.406: R102.1 32.7,74.3 33.02,73.98 IC101.2
LED-R
  Top 0.406: IC101.4 32.38,68.9 R101.1
LINKS
  Bottom 0.406: IC101.26 51.44,40.96 52.39,41.91 52.39,84.45 55.88,87.95 OK201.2
MAGNET
  Bottom 0.406: OK205.2 53.02,11.75 51.75,13.02 51.75,29.53 50.48,30.8 IC101.22
MISO  (via drill 0.5)
  Top 0.406: v37.47,61.28 v37.47,26.99 | SV101.1 47.31,11.43 IC102.2
  Bottom 0.406: IC101.7 v37.47,61.28 | v37.47,26.99 42.23,26.99 | 42.23,26.99 42.23,20.32 40.96,19.05 IC104.15 | SV101.1 49.53,10.16 50.48,11.11 50.48,26.04 49.53,26.99 42.23,26.99
MOSI  (via drill 0.5)
  Top 0.406: v38.42,63.82 38.42,26.04 39.69,24.77 v39.69,20.64
  Bottom 0.406: IC101.6 v38.42,63.82 | v39.69,20.64 39.69,20.32 38.42,19.05 IC104.14 38.42,8.26 40.64,6.03 | 40.64,6.03 40.96,5.71 IC102.5 | SV101.4 44.13,7.62 42.86,8.89 41.27,8.89 40.64,8.26 40.64,6.03
N$1  (via drill 0.5)
  Top 0.406: v34.61,18.73 45.4,18.73 48.58,21.91 IC104.1
  Bottom 0.406: IC105.1 34.61,13.97 v34.61,18.73
N$2
  Top 0.406: IC104.2 46.04,20.95 44.77,19.68 31.75,19.68 29.53,17.46 29.53,13.97 IC105.4
N$3
  Bottom 0.406: R106.1 19.37,14.29 20.32,13.34 21.59,13.34 22.23,12.7 OK101.3
N$4  (via drill 0.5)
  Top 0.406: v22.86,47.94 v22.86,29.84 | J101.3 18.1,12.38 v20.64,14.92
  Bottom 0.406: R109.2 v22.86,47.94 | v22.86,29.84 22.86,28.57 26.67,24.77 26.67,19.68 24.77,17.78 OK101.1 24.77,15.56 24.13,14.92 v20.64,14.92
N$5
  Top 0.406: R110.1 24.13,65.09 27.3,68.26 D104.C
N$6
  Bottom 0.813: C105.+ 43.18,83.5 39.05,87.63 30.16,87.63 D102.C 28.57,87.95 27.3,86.68 V101.IN
N$7
  Top 0.61: OK201.1 57.15,90.49 56.2,91.44 R216.2
N$9  (via drill 0.5)
  Top 0.406: R101.2 16.51,71.44 10.79,77.15 v10.48,77.15
  Bottom 0.406: v10.48,77.15 D101.AR
N$10
  Bottom 0.813: R207.1 T201.G OK201.4
N$11
  Top 0.813: R206.1 64.77,94.93 67.63,92.08 OK201.6
N$12
  Top 0.61: OK202.1 57.15,70.17 56.2,71.12 R217.2
N$13  (via drill 0.5)
  Top 0.406: R102.2 18.73,74.3 10.79,82.23 v10.48,82.23
  Bottom 0.406: v10.48,82.23 D101.AG
N$15
  Top 0.813: R201.2 76.83,84.45 79.06,86.68 C201.1
N$17
  Bottom 0.813: R209.1 T202.G OK202.4
N$18
  Top 0.813: R208.1 64.45,74.61 67.63,71.44 OK202.6
N$20
  Top 0.813: R202.2 76.83,64.14 79.06,66.36 C202.1
N$21
  Top 0.61: OK203.1 57.15,52.39 56.2,53.34 R218.2
N$23
  Bottom 0.813: R211.1 T203.G OK203.4
N$24
  Top 0.813: R210.1 64.77,56.83 67.63,53.98 OK203.6
N$26
  Top 0.813: R203.2 76.83,46.35 79.06,48.58 C203.1
N$27
  Top 0.61: OK204.1 57.15,34.61 56.2,35.56 R219.2
N$29
  Bottom 0.813: R213.1 T204.G OK204.4
N$30
  Top 0.813: R212.1 64.77,39.05 67.63,36.2 OK204.6
N$32
  Top 0.813: R204.2 76.83,28.89 78.74,30.8 C204.1
N$33
  Top 0.61: OK205.1 57.15,14.29 56.2,15.24 R220.2
N$35
  Bottom 0.813: R215.1 T205.G OK205.4
N$36
  Top 0.813: R214.1 64.77,18.73 67.63,15.88 OK205.6
N$38
  Top 0.813: R205.2 76.83,8.26 79.06,10.48 C205.1
P10
  Bottom 0.406: X101.1 6.67,71.76 13.65,64.77 13.65,49.21 18.1,44.77 30.16,44.77 31.43,43.5 IC101.14
P11
  Bottom 0.406: X101.2 6.99,68.26 12.7,62.55 12.7,48.9 20.64,40.96 IC101.15
P12
  Bottom 0.406: X101.3 7,64.76 11.75,60.01 11.75,48.58 21.91,38.42 IC101.16
P13
  Bottom 0.406: IC101.17 26.35,35.88 26.04,36.2 22.86,36.2 10.79,48.26 10.79,57.47 6.99,61.28 5.32,61.28 X101.4
P14
  Bottom 0.406: X101.5 7.01,57.76 9.84,54.93 9.84,47.94 22.54,35.24 25.72,35.24 27.62,33.34 IC101.18
P15
  Bottom 0.406: X101.6 7.02,54.26 8.89,52.39 8.89,47.62 22.23,34.29 25.4,34.29 28.89,30.8 IC101.19
P16
  Bottom 0.406: X101.7 7.03,50.76 7.94,49.85 7.94,47.31 21.91,33.34 25.08,33.34 28.57,29.84 30.48,29.84 32.07,28.26 IC101.20
P17
  Bottom 0.406: X101.8 6.72,47.26 21.59,32.38 24.77,32.38 26.04,31.11 26.04,27.94 26.99,26.99 34.92,26.99 36.2,28.26 IC101.21
PLUGGED  (via drill 0.5)
  Top 0.406: R111.1 R110.2 34.92,65.09 35.56,65.72 v35.56,73.03
  Bottom 0.406: IC101.39 36.51,73.98 v35.56,73.03
Q-CLK
  Top 0.406: IC101.13 30.8,43.18 30.8,28.26 | 30.8,28.26 IC104.8 | 30.8,28.26 QG101.8
RAUF
  Bottom 0.406: OK203.2 56.2,49.85 54.93,48.58 54.93,38.42 52.39,35.88 IC101.24
RECHTS
  Bottom 0.406: IC101.25 52.39,38.42 53.66,39.69 53.66,66.04 55.24,67.63 OK202.2
RUNTER
  Bottom 0.406: IC101.23 53.02,33.34 54.29,32.07 OK204.2
SCK  (via drill 0.5)
  Top 0.406: v36.51,58.74 36.51,26.04 37.15,25.4 v37.15,20.64 | IC102.6 43.5,8.89 SV101.3
  Bottom 0.406: IC101.8 v36.51,58.74 | v37.15,20.64 37.15,20.32 35.88,19.05 IC104.13 35.88,15.24 37.15,13.97 37.15,8.26 38.73,6.67 38.73,3.81 39.37,3.17 42.86,3.17 43.5,3.81 IC102.6
SPG
  Bottom 0.61: R107.2 R108.1 41.27,78.74 43.5,76.52 IC101.40
TRACK-0
  Bottom 0.813: J102.1 9.21,33.34 9.21,16.51 J101.1
TRACK-B
  Top 0.813: J102.2 13.34,34.92 11.43,36.83 9.84,36.83 9.21,36.2 9.21,19.68 13.34,15.56 J101.2
V-NETZTEIL  (via drill 0.5)
  Top 0.406: v16.83,73.03 17.14,72.71 23.5,72.71 24.13,72.07 24.13,68.9 23.5,68.26 D104.A
  Top 0.813: D103.A 21.59,93.34 17.14,88.9 v16.19,88.9 13.65,91.44 7.62,91.44 X102.2
  Bottom 0.406: v16.19,88.9 16.19,73.66 v16.83,73.03

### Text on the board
Bottom: bottom | 17.11.2019 | MBCAN-Projekt | (c) Dr.-Ing. Th. Wiesner | mbc87.brd
tNames: HW: 19.11.17 | +18V | DC | AC | +18V | (c) Dr.-Ing. Th. Wiesner | MBCAN-Projekt | 0 | IN | MAG | OUT | mbc-87
bNames: 26.10.2019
